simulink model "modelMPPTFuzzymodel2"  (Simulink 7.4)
settings: Solver=ode1  SolverMode=SingleTasking  StartTime=0.0  StopTime=5  FixedStep=1e-4  MaxStep=1e-5
libraries: fuzblock x1, simulink x1

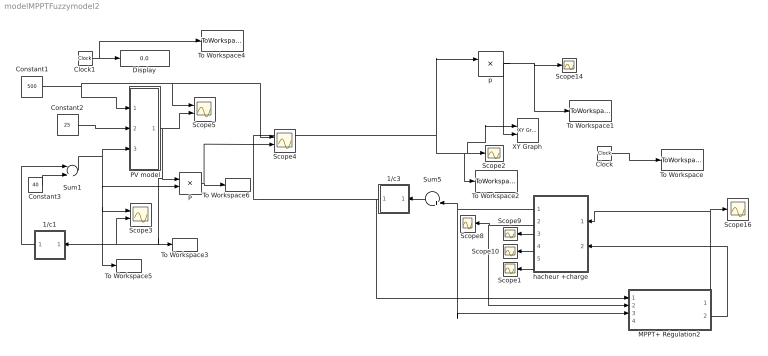
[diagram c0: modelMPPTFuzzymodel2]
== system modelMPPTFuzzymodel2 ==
  1/c1 : Subsystem
  1/c3 : Subsystem
  Clock : Clock
  Clock1 : Clock
  Constant1 : Constant  Value=500  OutDataType=sfix(16)  OutScaling=2^0
  Constant2 : Constant  Value=25  OutDataType=sfix(16)  OutScaling=2^0
  Constant3 : Constant  Value=40  OutDataType=sfix(16)  OutScaling=2^0
  Display : Display
  MPPT+ Régulation2 : Subsystem
  P : Product  OutDataType=sfix(16)  OutScaling=2^0
  PV model : Subsystem  mask{p1=0.00345, p2=0.0058e-3, p3=-0.0336e-3, p4=31.2367, Eg=1.76e-19, k=1.38e-23, e0=1.6e-19, a=1, ns=72, rs=0.9225, rsh=235.1551, Eref=1000, Tjref=298}
  Scope{1..2,8..10,14,16} (7 alike) : Scope
  Scope3 : Scope  NumInputPorts=2
  Scope4 : Scope  NumInputPorts=2
  Scope5 : Scope  NumInputPorts=2
  Sum1 : Sum  Inputs=|+-  OutDataType=sfix(16)  OutScaling=2^0
  Sum5 : Sum  Inputs=|+-  OutDataType=sfix(16)  OutScaling=2^0
  To Workspace : ToWorkspace  VariableName=t  SampleTime=-1  SaveFormat=Array
  To Workspace1 : ToWorkspace  VariableName=P  SampleTime=-1  SaveFormat=Array
  To Workspace2 : ToWorkspace  VariableName=V  SampleTime=-1  SaveFormat=Array
  To Workspace3 : ToWorkspace  VariableName=i  SampleTime=-1  SaveFormat=Array
  To Workspace4 : ToWorkspace  VariableName=t1  SampleTime=-1  SaveFormat=Array
  To Workspace5 : ToWorkspace  VariableName=v  SampleTime=-1  SaveFormat=Array
  To Workspace6 : ToWorkspace  VariableName=p  SampleTime=-1  SaveFormat=Array
  XY Graph : simulink/Sinks/XY Graph  SystemSampleTime=-1  xmin=0  xmax=50  ymin=0  ymax=120  st=-1
  hacheur +charge : Subsystem
  p : Product  OutDataType=sfix(16)  OutScaling=2^0
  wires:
  1/c3/1(Vdc) -> MPPT+ Régulation2/1(vpv), p/1, Scope2/1, XY Graph/1, To Workspace2/1
  hacheur +charge/3(iCH) -> Scope9/1
  hacheur +charge/4(Pch) -> Scope10/1
  hacheur +charge/2(Vch) -> Scope8/1, MPPT+ Régulation2/2(vch)
  MPPT+ Régulation2/1(1-alpha) -> hacheur +charge/1(" 1-alpha"), Scope16/1
  MPPT+ Régulation2/2(VPV1) -> hacheur +charge/2(vpv)
  p/1 -> Scope14/1, To Workspace1/1, XY Graph/2
  hacheur +charge/5(iL'1) -> Scope1/1
  hacheur +charge/1(iL) -> Sum5/2, MPPT+ Régulation2/3(il)
  Clock/1 -> To Workspace/1
  Sum5/1 -> 1/c3/1(Idc)
  ? -> MPPT+ Régulation2/4(ipv), Sum5/1, p/2
  Constant2/1 -> PV model/2(Ta)
  Constant3/1 -> Sum1/2
  Sum1/1 -> PV model/3(V), P/2, To Workspace5/1, Scope3/1
  P/1 -> Scope4/2, To Workspace6/1
  Clock1/1 -> Display/1, To Workspace4/1
  PV model/1(I1) -> Scope5/2, P/1, To Workspace3/1, Scope3/2, 1/c1/1(Idc)
  Constant1/1 -> PV model/1(Es), Scope5/1, Scope4/1
  1/c1/1(Vdc) -> Sum1/1

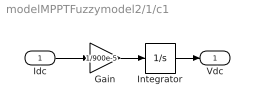
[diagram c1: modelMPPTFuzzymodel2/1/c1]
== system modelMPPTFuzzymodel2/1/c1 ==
  Idc : Inport  OutDataType=sfix(16)  OutScaling=2^0
  Gain : Gain  Gain=1/900e-5  ParameterDataType=sfix(16)  ParameterScaling=2^0  OutDataType=sfix(16)  OutScaling=2^0
  Integrator : Integrator
  Vdc : Outport
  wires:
  Gain/1 -> Integrator/1
  Idc/1 -> Gain/1
  Integrator/1 -> Vdc/1

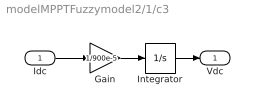
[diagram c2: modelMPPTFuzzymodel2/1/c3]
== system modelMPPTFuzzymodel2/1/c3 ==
  Idc : Inport  OutDataType=sfix(16)  OutScaling=2^0
  Gain : Gain  Gain=1/900e-5  ParameterDataType=sfix(16)  ParameterScaling=2^0  OutDataType=sfix(16)  OutScaling=2^0
  Integrator : Integrator
  Vdc : Outport
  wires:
  Gain/1 -> Integrator/1
  Idc/1 -> Gain/1
  Integrator/1 -> Vdc/1

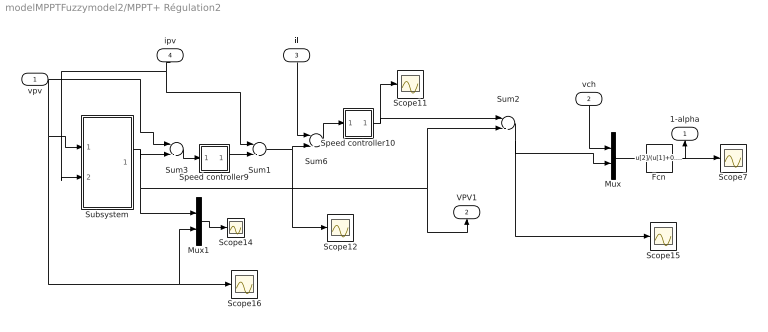
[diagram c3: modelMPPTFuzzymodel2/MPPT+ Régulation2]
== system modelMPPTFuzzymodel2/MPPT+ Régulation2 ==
  vpv : Inport  OutDataType=sfix(16)  OutScaling=2^0
  vch : Inport  Port=2  OutDataType=sfix(16)  OutScaling=2^0
  il : Inport  Port=3  OutDataType=sfix(16)  OutScaling=2^0
  ipv : Inport  Port=4  OutDataType=sfix(16)  OutScaling=2^0
  Fcn : Fcn  Expr=u[2]/(u[1]+0.1)
  Mux : Mux  Inputs=2
  Mux1 : Mux  Inputs=2
  Scope{7,11..12,14..16} (6 alike) : Scope
  Speed controller10 : Subsystem  mask{Kp2=0.01, Ki2=0.1963}
      mask prompts: Kp2 "Proportional gain (Kp)"; Ki2 "Integral gain (Ki)"
      mask help: Proportional-Integral Speed Controller
  Speed controller9 : Subsystem  mask{Kp2=7, Ki2=33.62}
      mask prompts: Kp2 "Proportional gain (Kp)"; Ki2 "Integral gain (Ki)"
      mask help: Proportional-Integral Speed Controller
  Subsystem : Subsystem
  Sum{1..3,6} (4 alike) : Sum  Inputs=|-+  OutDataType=sfix(16)  OutScaling=2^0
  1-alpha : Outport
  VPV1 : Outport  Port=2
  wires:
  Mux1/1 -> Scope14/1
  Subsystem/1(Vref) -> Mux1/1, VPV1/1, Sum2/2, Sum3/2
  Speed controller9/1(Ura) -> Sum1/2
  vpv/1 -> Sum3/1, Scope16/1, Mux1/2, Subsystem/1(Vpv)
  Sum1/1 -> Scope12/1, Sum6/2
  vch/1 -> Mux/1
  Sum2/1 -> Mux/2, Scope15/1
  Fcn/1 -> 1-alpha/1, Scope7/1
  Mux/1 -> Fcn/1
  Speed controller10/1(Ura) -> Sum2/1, Scope11/1
  Sum6/1 -> Speed controller10/1(Ia)
  ipv/1 -> Sum1/1, Subsystem/2(Ipv)
  Sum3/1 -> Speed controller9/1(Ia)
  il/1 -> Sum6/1

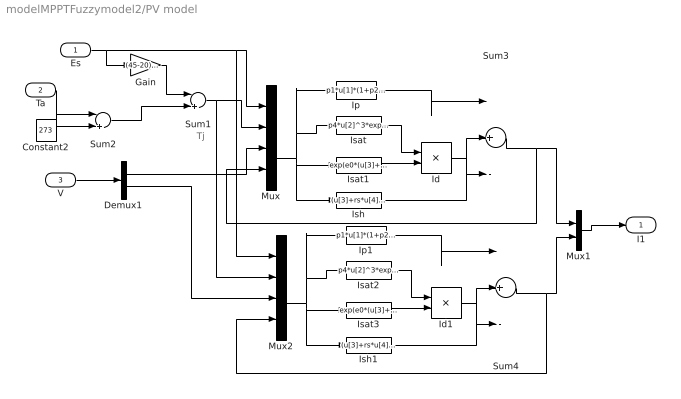
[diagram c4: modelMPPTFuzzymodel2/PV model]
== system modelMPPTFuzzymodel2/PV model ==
  note: Tj
  Es : Inport  OutDataType=sfix(16)  OutScaling=2^0
  Ta : Inport  Port=2  OutDataType=sfix(16)  OutScaling=2^0
  V : Inport  Port=3  OutDataType=sfix(16)  OutScaling=2^0
  Constant2 : Constant  Value=273  OutDataType=sfix(16)  OutScaling=2^0
  Demux1 : Demux  Outputs=2
  Gain : Gain  Gain=(45-20)/800  ParameterDataType=sfix(16)  ParameterScaling=2^0  OutDataType=sfix(16)  OutScaling=2^0
  Id : Product  OutDataType=sfix(16)  OutScaling=2^0
  Id1 : Product  OutDataType=sfix(16)  OutScaling=2^0
  Ip : Fcn  Expr=p1*u[1]*(1+p2*(u[1]-Eref)+p3*(u[2]-Tjref))
  Ip1 : Fcn  Expr=p1*u[1]*(1+p2*(u[1]-Eref)+p3*(u[2]-Tjref))
  Isat : Fcn  Expr=p4*u[2]^3*exp(-Eg/(k*u[2]))
  Isat1 : Fcn  Expr=exp(e0*(u[3]+rs*u[4])/(a*ns*k*u[2]))-1
  Isat2 : Fcn  Expr=p4*u[2]^3*exp(-Eg/(k*u[2]))
  Isat3 : Fcn  Expr=exp(e0*(u[3]+rs*u[4])/(a*ns*k*u[2]))-1
  Ish : Fcn  Expr=(u[3]+rs*u[4])/rsh
  Ish1 : Fcn  Expr=(u[3]+rs*u[4])/rsh
  Mux : Mux
  Mux1 : Mux  Inputs=2
  Mux2 : Mux
  Sum1 : Sum  Inputs=|++  OutDataType=sfix(16)  OutScaling=2^0
  Sum2 : Sum  Inputs=|++  OutDataType=sfix(16)  OutScaling=2^0
  Sum3 : Sum  Inputs=|+--  OutDataType=sfix(16)  OutScaling=2^0
  Sum4 : Sum  Inputs=|+--  OutDataType=sfix(16)  OutScaling=2^0
  I1 : Outport
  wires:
  Es/1 -> Gain/1, Mux/1, Mux2/1
  Gain/1 -> Sum1/1
  Constant2/1 -> Sum2/2
  Isat/1 -> Id/1
  Isat1/1 -> Id/2
  Mux/1 -> Ip/1, Isat/1, Isat1/1, Ish/1
  Id/1 -> Sum3/2
  Ip/1 -> Sum3/1
  Ish/1 -> Sum3/3
  Sum3/1 -> Mux/4, Mux1/1
  Ta/1 -> Sum2/1
  V/1 -> Demux1/1
  Demux1/1 -> Mux/3
  Isat2/1 -> Id1/1
  Isat3/1 -> Id1/2
  Mux2/1 -> Ish1/1, Isat3/1, Isat2/1, Ip1/1
  Id1/1 -> Sum4/2
  Ip1/1 -> Sum4/1
  Ish1/1 -> Sum4/3
  Sum4/1 -> Mux2/4, Mux1/2
  Demux1/2 -> Mux2/3
  Mux1/1 -> I1/1
  Sum2/1 -> Sum1/2
  Sum1/1 -> Mux/2, Mux2/2

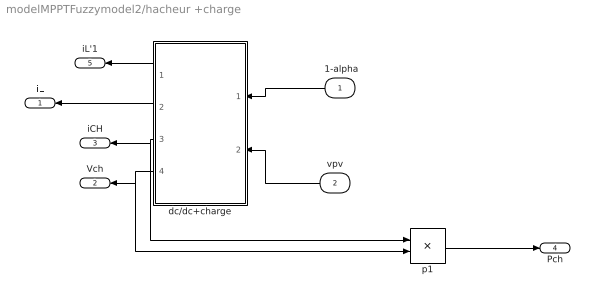
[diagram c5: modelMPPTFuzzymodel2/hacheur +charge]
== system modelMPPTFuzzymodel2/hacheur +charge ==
  " 1-alpha" : Inport  OutDataType=sfix(16)  OutScaling=2^0
  vpv : Inport  Port=2  OutDataType=sfix(16)  OutScaling=2^0
  dc/dc+charge : Subsystem
  p1 : Product  OutDataType=sfix(16)  OutScaling=2^0
  iL : Outport
  Vch : Outport  Port=2
  iCH : Outport  Port=3
  Pch : Outport  Port=4
  iL'1 : Outport  Port=5
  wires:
  vpv/1 -> dc/dc+charge/2(vcpv)
  dc/dc+charge/3(iCH) -> iCH/1, p1/1
  dc/dc+charge/4(Vch) -> Vch/1, p1/2
  p1/1 -> Pch/1
  dc/dc+charge/2(iL) -> iL/1
  " 1-alpha"/1 -> dc/dc+charge/1(1-alpha)
  dc/dc+charge/1(iL'1) -> iL'1/1

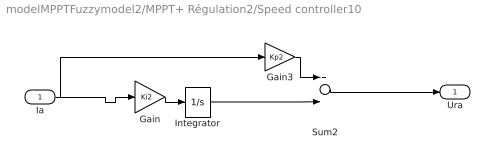
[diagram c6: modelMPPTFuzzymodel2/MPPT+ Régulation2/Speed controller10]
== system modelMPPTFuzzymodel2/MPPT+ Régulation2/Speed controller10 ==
  Ia : Inport  OutDataType=sfix(16)  OutScaling=2^0
  Gain : Gain  Gain=Ki2  ParameterDataType=sfix(16)  ParameterScaling=2^0  OutDataType=sfix(16)  OutScaling=2^0
  Gain3 : Gain  Gain=Kp2  ParameterDataType=sfix(16)  ParameterScaling=2^0  OutDataType=sfix(16)  OutScaling=2^0
  Integrator : Integrator  UpperSaturationLimit=30  LowerSaturationLimit=-30
  Sum2 : Sum  OutDataType=sfix(16)  OutScaling=2^0
  Ura : Outport  InitialOutput=0
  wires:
  Gain/1 -> Integrator/1
  Gain3/1 -> Sum2/1
  Sum2/1 -> Ura/1
  Integrator/1 -> Sum2/2
  Ia/1 -> Gain/1, Gain3/1

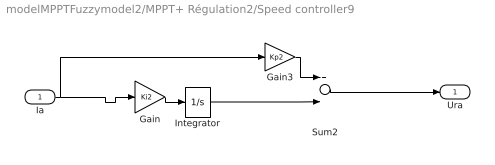
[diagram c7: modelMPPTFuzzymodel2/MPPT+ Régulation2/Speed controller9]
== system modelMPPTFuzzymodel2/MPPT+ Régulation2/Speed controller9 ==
  Ia : Inport  OutDataType=sfix(16)  OutScaling=2^0
  Gain : Gain  Gain=Ki2  ParameterDataType=sfix(16)  ParameterScaling=2^0  OutDataType=sfix(16)  OutScaling=2^0
  Gain3 : Gain  Gain=Kp2  ParameterDataType=sfix(16)  ParameterScaling=2^0  OutDataType=sfix(16)  OutScaling=2^0
  Integrator : Integrator  UpperSaturationLimit=30  LowerSaturationLimit=-30
  Sum2 : Sum  OutDataType=sfix(16)  OutScaling=2^0
  Ura : Outport  InitialOutput=0
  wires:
  Ia/1 -> Gain3/1, Gain/1
  Integrator/1 -> Sum2/2
  Sum2/1 -> Ura/1
  Gain3/1 -> Sum2/1
  Gain/1 -> Integrator/1

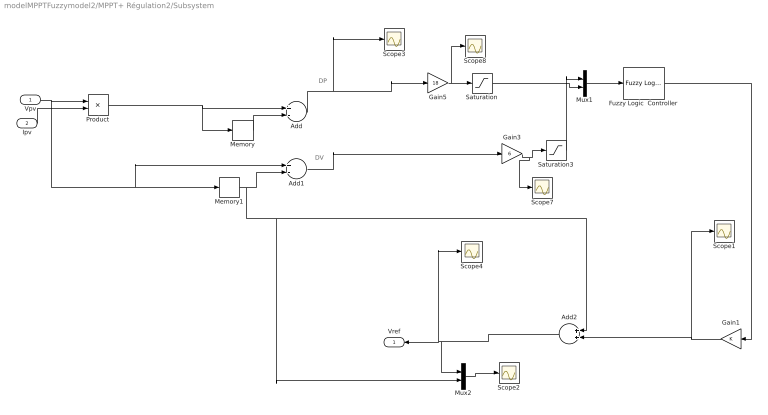
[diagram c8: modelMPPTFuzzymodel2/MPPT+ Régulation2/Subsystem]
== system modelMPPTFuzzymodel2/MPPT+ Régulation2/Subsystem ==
  note: DP
  note: DV
  Vpv : Inport
  Ipv : Inport  Port=2
  Add : Sum  Inputs=+-  OutDataType=sfix(16)  OutScaling=2^-10
  Add1 : Sum  Inputs=+-  OutDataType=sfix(16)  OutScaling=2^-10
  Add2 : Sum  OutDataType=sfix(16)  OutScaling=2^-10
  Fuzzy Logic  Controller : fuzblock/Fuzzy Logic  Controller  SystemSampleTime=-1  fis=SAMM
  Gain1 : Gain  ParameterDataType=sfix(16)  ParameterScaling=2^0  OutDataType=sfix(16)  OutScaling=2^0
  Gain3 : Gain  Gain=6  ParameterDataType=sfix(16)  ParameterScaling=2^0  OutDataType=sfix(16)  OutScaling=2^0
  Gain5 : Gain  Gain=18  ParameterDataType=sfix(16)  ParameterScaling=2^0  OutDataType=sfix(16)  OutScaling=2^0
  Memory : Memory
  Memory1 : Memory
  Mux1 : Mux  Inputs=2
  Mux2 : Mux  Inputs=2
  Product : Product  OutDataType=sfix(16)  OutScaling=2^0
  Saturation : Saturate  UpperLimit=1  LowerLimit=-1  OutDataType=sfix(16)  OutScaling=2^0
  Saturation3 : Saturate  UpperLimit=1  LowerLimit=-1  OutDataType=sfix(16)  OutScaling=2^0
  Scope{1..4,7..8} (6 alike) : Scope
  Vref : Outport  OutDataType=sfix(16)  OutScaling=2^0
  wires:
  Memory/1 -> Add/2
  Memory1/1 -> Add1/2, Add2/1, Mux2/2
  Fuzzy Logic  Controller/1 -> Gain1/1
  Add1/1 -> Gain3/1
  Product/1 -> Add/1, Memory/1
  Add/1 -> Scope3/1, Gain5/1
  Gain5/1 -> Scope8/1, Saturation/1
  Mux1/1 -> Fuzzy Logic  Controller/1
  Gain3/1 -> Scope7/1, Saturation3/1
  Gain1/1 -> Scope1/1, Add2/2
  Vpv/1 -> Memory1/1, Add1/1, Product/1
  Ipv/1 -> Product/2
  Saturation3/1 -> Mux1/1
  Saturation/1 -> Mux1/2
  Add2/1 -> Vref/1, Scope4/1, Mux2/1
  Mux2/1 -> Scope2/1

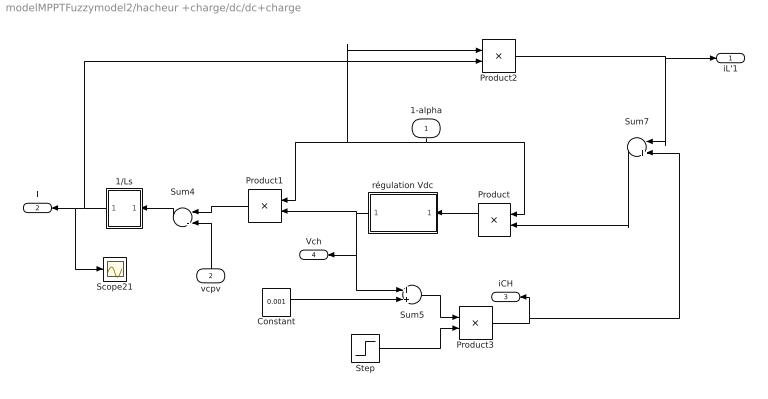
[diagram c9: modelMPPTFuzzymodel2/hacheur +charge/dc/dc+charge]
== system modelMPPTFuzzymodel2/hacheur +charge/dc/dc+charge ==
  1-alpha : Inport  OutDataType=sfix(16)  OutScaling=2^0
  vcpv : Inport  Port=2  OutDataType=sfix(16)  OutScaling=2^0
  1/Ls : Subsystem
  Constant : Constant  Value=0.001  OutDataType=sfix(16)  OutScaling=2^0
  Product : Product  OutDataType=sfix(16)  OutScaling=2^0
  Product1 : Product  OutDataType=sfix(16)  OutScaling=2^0
  Product2 : Product  OutDataType=sfix(16)  OutScaling=2^0
  Product3 : Product  Inputs=/*  OutDataType=sfix(16)  OutScaling=2^0
  Scope21 : Scope
  Step : Step  Before=70  After=70  SampleTime=0
  Sum4 : Sum  Inputs=|-+  OutDataType=sfix(16)  OutScaling=2^0
  Sum5 : Sum  OutDataType=sfix(16)  OutScaling=2^0
  Sum7 : Sum  Inputs=|+-  OutDataType=sfix(16)  OutScaling=2^0
  régulation Vdc : Subsystem
  iL'1 : Outport
  iL : Outport  Port=2
  iCH : Outport  Port=3
  Vch : Outport  Port=4
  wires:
  régulation Vdc/1(Vdc) -> Product1/2, Vch/1, Sum5/1
  Sum7/1 -> Product/2
  1-alpha/1 -> Product/1, Product1/1, Product2/1
  Sum4/1 -> 1/Ls/1(ul)
  vcpv/1 -> Sum4/2
  Product/1 -> régulation Vdc/1(Idc)
  Product1/1 -> Sum4/1
  1/Ls/1(il) -> iL/1, Scope21/1, Product2/2
  Product2/1 -> Sum7/1, iL'1/1
  Step/1 -> Product3/2
  Product3/1 -> iCH/1, Sum7/2
  Sum5/1 -> Product3/1
  Constant/1 -> Sum5/2

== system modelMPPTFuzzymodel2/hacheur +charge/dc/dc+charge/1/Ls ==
  ul : Inport  OutDataType=sfix(16)  OutScaling=2^0
  Gain : Gain  Gain=1/0.66e-5  ParameterDataType=sfix(16)  ParameterScaling=2^0  OutDataType=sfix(16)  OutScaling=2^0
  Integrator : Integrator
  il : Outport
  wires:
  Integrator/1 -> il/1
  ul/1 -> Gain/1
  Gain/1 -> Integrator/1

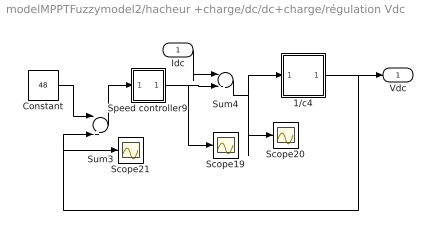
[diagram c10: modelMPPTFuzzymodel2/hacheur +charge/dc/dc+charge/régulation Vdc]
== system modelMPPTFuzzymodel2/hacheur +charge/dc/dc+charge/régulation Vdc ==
  Idc : Inport  OutDataType=sfix(16)  OutScaling=2^0
  1/c4 : Subsystem
  Constant : Constant  Value=48  OutDataType=sfix(16)  OutScaling=2^0
  Scope19 : Scope
  Scope20 : Scope
  Scope21 : Scope
  Speed controller9 : Subsystem  mask{Kp2=98, Ki2=220}
      mask prompts: Kp2 "Proportional gain (Kp)"; Ki2 "Integral gain (Ki)"
      mask help: Proportional-Integral Speed Controller
  Sum3 : Sum  Inputs=|+-  OutDataType=sfix(16)  OutScaling=2^0
  Sum4 : Sum  Inputs=|-+  OutDataType=sfix(16)  OutScaling=2^0
  Vdc : Outport
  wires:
  Sum3/1 -> Speed controller9/1(Ia)
  Constant/1 -> Sum3/1
  Idc/1 -> Sum4/1
  1/c4/1(Vdc) -> Vdc/1, Sum3/2, Scope21/1
  Speed controller9/1(Ura) -> Sum4/2, Scope19/1
  Sum4/1 -> 1/c4/1(Idc), Scope20/1

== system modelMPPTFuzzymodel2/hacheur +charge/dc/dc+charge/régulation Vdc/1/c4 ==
  Idc : Inport  OutDataType=sfix(16)  OutScaling=2^0
  Gain : Gain  Gain=1/900e-5  ParameterDataType=sfix(16)  ParameterScaling=2^0  OutDataType=sfix(16)  OutScaling=2^0
  Integrator : Integrator
  Vdc : Outport
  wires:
  Gain/1 -> Integrator/1
  Idc/1 -> Gain/1
  Integrator/1 -> Vdc/1

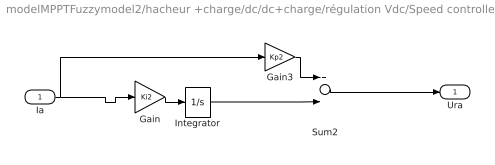
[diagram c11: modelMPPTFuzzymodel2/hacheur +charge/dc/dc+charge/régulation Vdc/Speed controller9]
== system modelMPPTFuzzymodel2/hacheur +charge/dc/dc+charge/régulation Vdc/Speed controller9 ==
  Ia : Inport  OutDataType=sfix(16)  OutScaling=2^0
  Gain : Gain  Gain=Ki2  ParameterDataType=sfix(16)  ParameterScaling=2^0  OutDataType=sfix(16)  OutScaling=2^0
  Gain3 : Gain  Gain=Kp2  ParameterDataType=sfix(16)  ParameterScaling=2^0  OutDataType=sfix(16)  OutScaling=2^0
  Integrator : Integrator  UpperSaturationLimit=30  LowerSaturationLimit=-30
  Sum2 : Sum  OutDataType=sfix(16)  OutScaling=2^0
  Ura : Outport  InitialOutput=0
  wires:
  Ia/1 -> Gain3/1, Gain/1
  Integrator/1 -> Sum2/2
  Sum2/1 -> Ura/1
  Gain3/1 -> Sum2/1
  Gain/1 -> Integrator/1
